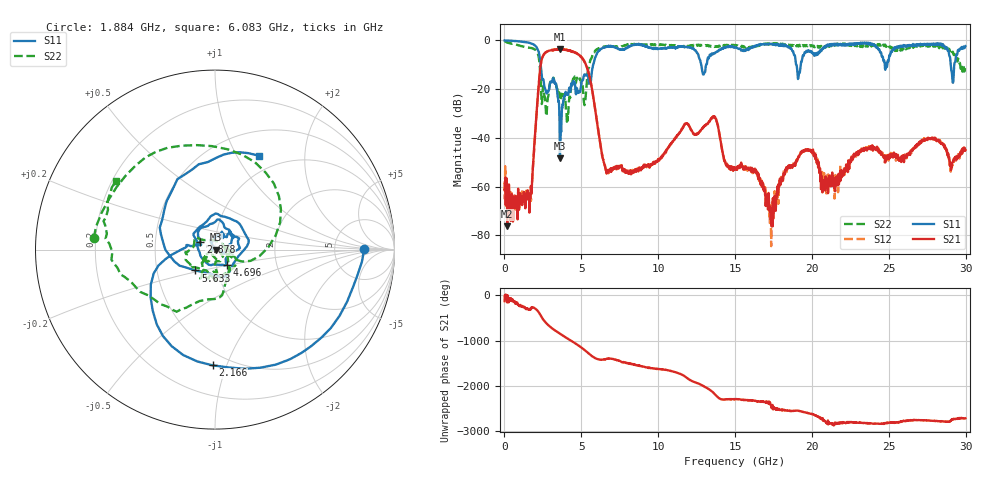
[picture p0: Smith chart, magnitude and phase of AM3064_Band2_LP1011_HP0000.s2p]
# Hz S DB R 50.0
!freq dBS11 angS11 dBS21 angS21 dBS12 angS12 dBS22 angS22
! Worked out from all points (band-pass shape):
!   1600 points, 10 MHz to 29.98 GHz, reference 50 ohm
!   highest |S21| = -3.60 dB at 3.59 GHz (marker M1); lowest = -76.4 dB at 178.7 MHz (marker M2)
!   |S21| within 3 dB of the highest: 2.492 GHz to 4.951 GHz (2.459 GHz wide, 66.1 % of centre)
!   lowest |S11| = -48.4 dB at 3.609 GHz (marker M3), VSWR 1.01, Z = 50.4 - j0.125 ohm
!   |S11| at or under -10 dB: 2.357 GHz to 5.768 GHz (3.411 GHz wide, 84 % of centre); 12.8 GHz to 13.12 GHz (319.8 MHz wide, 2.47 % of centre); 18.98 GHz to 19.27 GHz (288.9 MHz wide, 1.51 % of centre)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
!   |S22| runs from -33.4 to -0.3 dB; largest |S21 - S12| = 0.019
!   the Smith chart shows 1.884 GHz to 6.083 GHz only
!   S11 on the Smith chart (normalised r, x): 1.884 GHz: 11, +0; 2.166 GHz: 0.41, -0.90; 2.878 GHz: 0.85, +0.07; 4.696 GHz: 1.12, -0.19; 5.633 GHz: 0.78, -0.19; 6.083 GHz: 0.79, +1.24
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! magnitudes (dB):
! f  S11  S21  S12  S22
! 10 MHz  0.0  -61.3  -57.9  -0.3
! 178.7 MHz  -0.1  -76.4  -69.9  -0.9
! 1.622 GHz  -1.0  -70.7  -66.5  -3.0
! 1.884 GHz  -1.6  -49.0  -48.9  -3.4
! 2.166 GHz  -3.8  -23.3  -23.3  -5.4
! 2.878 GHz  -20.7  -4.3  -4.2  -21.4
! 3.59 GHz  -37.4  -3.6  -3.7  -22.6
! 3.609 GHz  -48.4  -3.9  -3.7  -22.9
! 4.696 GHz  -19.5  -5.4  -5.4  -15.7
! 5.015 GHz  -16.9  -7.1  -6.9  -18.3
! 5.633 GHz  -15.9  -17.8  -17.8  -7.7
! 6.083 GHz  -4.8  -36.1  -36.1  -3.5
! 6.702 GHz  -2.6  -54.2  -53.9  -2.5
! 10 GHz  -3.4  -48.8  -48.7  -1.8
! 13.6 GHz  -5.2  -31.6  -31.3  -2.5
! 15 GHz  -2.6  -52.4  -52.6  -1.9
! 17.37 GHz  -1.5  -69.8  -71.8  -1.2
! 19.99 GHz  -4.6  -46.0  -45.5  -2.0
! 20.91 GHz  -2.2  -58.7  -58.3  -2.4
! 25 GHz  -7.9  -47.5  -49.1  -2.2
! 29.18 GHz  -17.4  -49.8  -49.9  -4.8
! 29.98 GHz  -2.4  -45.1  -45.2  -10.3
